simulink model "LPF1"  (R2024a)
settings: Solver=ode45  StartTime=0.0  StopTime=0.5  MaxStep=1e-5  RelTol=1e-5  EnableMultiTasking=on
libraries: simulink x1

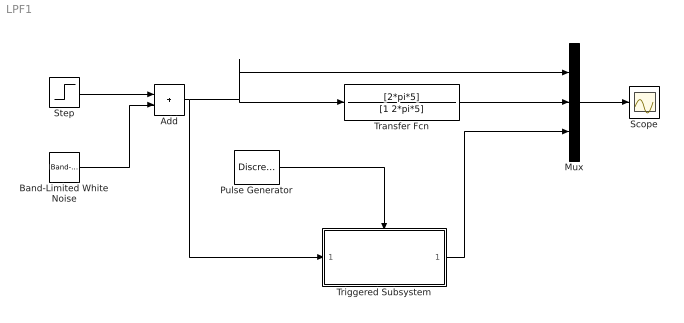
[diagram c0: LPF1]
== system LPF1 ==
  Add : Sum
  Band-Limited White Noise : simulink/Sources/Band-Limited White Noise  Cov=1E-9  Ts=0.00001  seed=[23341]
  Mux : Mux  Inputs=3
  Pulse Generator : DiscretePulseGenerator  PulseType=Time based  Period=0.0001  PulseWidth=50
  Scope : Scope
  Step : Step  Time=0.05  SampleTime=0
  Transfer Fcn : TransferFcn  Numerator=[2*pi*5]  Denominator=[1 2*pi*5]
  Triggered Subsystem : Subsystem  TreatAsAtomicUnit=on
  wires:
  Add/1 -> Triggered Subsystem/1(In1), Transfer Fcn/1, Mux/1
  Mux/1 -> Scope/1
  Pulse Generator/1 -> Triggered Subsystem/Trigger
  Step/1 -> Add/1
  Band-Limited White Noise/1 -> Add/2
  Transfer Fcn/1 -> Mux/2
  Triggered Subsystem/1(Out1) -> Mux/3

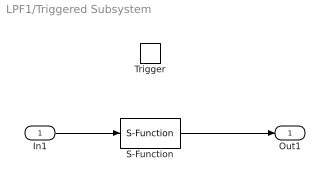
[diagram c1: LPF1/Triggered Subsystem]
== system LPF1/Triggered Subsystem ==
  In1 : Inport
  Trigger : TriggerPort  VariantControl=(inherit)
  S-Function : S-Function  FunctionName=controller  SFunctionDeploymentMode=off  EnableBusSupport=off
  Out1 : Outport
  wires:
  In1/1 -> S-Function/1
  S-Function/1 -> Out1/1
